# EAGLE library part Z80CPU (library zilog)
Z80 FAMILY DEVICE
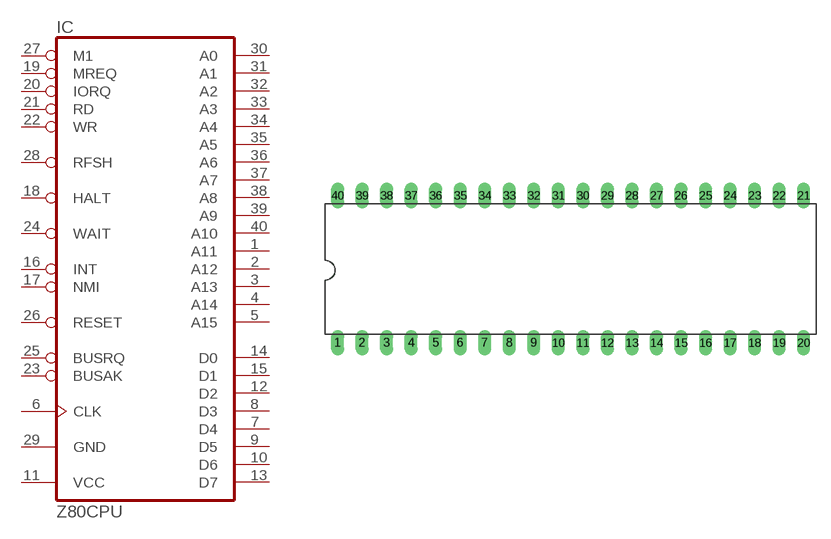
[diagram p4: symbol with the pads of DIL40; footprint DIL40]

Designator prefix IC

## Z80CPU  [DIL40]
1  A11  out
2  A12  out
3  A13  out
4  A14  out
5  A15  out
6  CLK  in
7  D4
8  D3
9  D5
10  D6
11  VCC  pwr
12  D2
13  D7
14  D0
15  D1
16  INT  in
17  NMI  in
18  HALT  out
19  MREQ  out
20  IORQ  out
21  RD  out
22  WR  out
23  BUSAK  out
24  WAIT  in
25  BUSRQ  in
26  RESET  in
27  M1  out
28  RFSH  out
29  GND  pwr
30  A0  out
31  A1  out
32  A2  out
33  A3  out
34  A4  out
35  A5  out
36  A6  out
37  A7  out
38  A8  out
39  A9  out
40  A10  out

## Footprint DIL40 (pad centres in mm)
Dual In Line Package
drill 0.813 long: 1 -24.13,-7.62; 2 -21.59,-7.62; 3 -19.05,-7.62; 4 -16.51,-7.62; 5 -13.97,-7.62; 6 -11.43,-7.62; 7 -8.89,-7.62; 8 -6.35,-7.62; 9 -3.81,-7.62; 10 -1.27,-7.62; 11 1.27,-7.62; 12 3.81,-7.62; 13 6.35,-7.62; 14 8.89,-7.62; 15 11.43,-7.62; 16 13.97,-7.62; 17 16.51,-7.62; 18 19.05,-7.62; 19 21.59,-7.62; 20 24.13,-7.62; 21 24.13,7.62; 22 21.59,7.62; 23 19.05,7.62; 24 16.51,7.62; 25 13.97,7.62; 26 11.43,7.62; 27 8.89,7.62; 28 6.35,7.62; 29 3.81,7.62; 30 1.27,7.62; 31 -1.27,7.62; 32 -3.81,7.62; 33 -6.35,7.62; 34 -8.89,7.62; 35 -11.43,7.62; 36 -13.97,7.62; 37 -16.51,7.62; 38 -19.05,7.62; 39 -21.59,7.62; 40 -24.13,7.62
